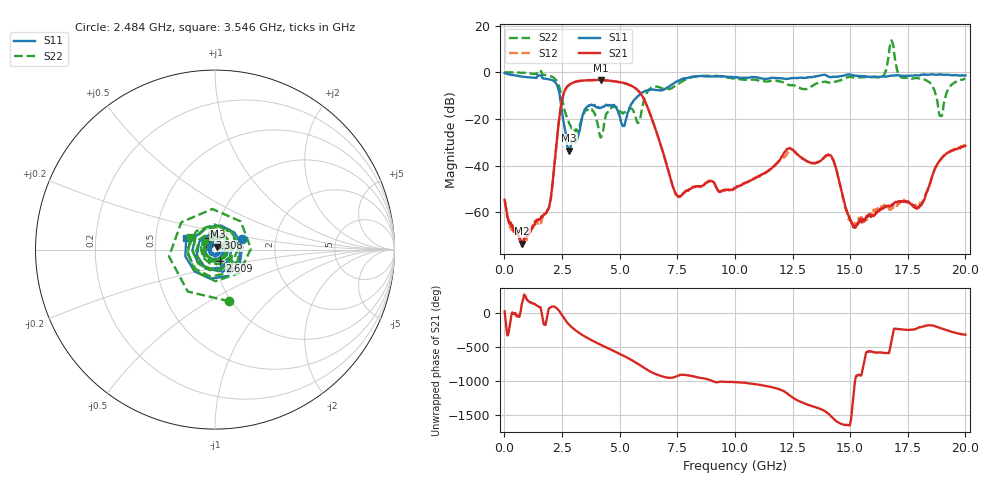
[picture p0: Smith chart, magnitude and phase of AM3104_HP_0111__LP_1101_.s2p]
!Created with skrf (http://scikit-rf.org).
# Hz S RI R 50.0
!freq ReS11 ImS11 ReS21 ImS21 ReS12 ImS12 ReS22 ImS22
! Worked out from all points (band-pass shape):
!   1601 points, 10 MHz to 20 GHz, reference 50 ohm
!   highest |S21| = -3.27 dB at 4.183 GHz (marker M1); lowest = -73.5 dB at 772.1 MHz (marker M2)
!   |S21| within 3 dB of the highest: 2.721 GHz to 5.594 GHz (2.873 GHz wide, 69.1 % of centre)
!   lowest |S11| = -33.7 dB at 2.809 GHz (marker M3), VSWR 1.04, Z = 51.3 + j1.65 ohm
!   |S11| at or under -10 dB: 2.401 GHz to 5.818 GHz (3.417 GHz wide, 83.1 % of centre)
!   |S22| runs from -28.0 to 13.6 dB; largest |S21 - S12| = 0.07
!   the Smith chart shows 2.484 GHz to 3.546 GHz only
!   S11 on the Smith chart (normalised r, x): 2.484 GHz: 1.34, +0.17; 2.609 GHz: 1.04, -0.13; 3.308 GHz: 0.93, +0.12; 3.546 GHz: 0.72, +0.09
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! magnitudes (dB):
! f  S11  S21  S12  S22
! 10 MHz  -0.4  -54.7  -55.3  0.0
! 772.1 MHz  -1.9  -73.5  -74.6  -0.2
! 1.922 GHz  -3.0  -58.3  -58.3  -1.4
! 2.484 GHz  -15.8  -12.8  -12.8  -10.5
! 2.609 GHz  -23.5  -8.1  -8.1  -16.2
! 2.809 GHz  -33.7  -5.4  -5.5  -21.9
! 3.308 GHz  -22.7  -3.7  -3.7  -21.4
! 3.346 GHz  -20.7  -3.6  -3.7  -20.2
! 3.546 GHz  -15.3  -3.5  -3.5  -16.3
! 4.183 GHz  -15.3  -3.3  -3.3  -28.0
! 5.157 GHz  -22.9  -4.5  -4.6  -17.6
! 5.795 GHz  -10.3  -7.8  -7.8  -21.8
! 6.682 GHz  -7.7  -28.1  -28.1  -6.3
! 7.506 GHz  -3.9  -52.9  -53.1  -5.2
! 10.01 GHz  -2.3  -49.8  -49.7  -2.9
! 13.34 GHz  -2.2  -39.0  -39.0  -6.0
! 14.2 GHz  -2.1  -36.4  -36.6  -4.5
! 15.16 GHz  -1.3  -66.5  -64.6  -2.2
! 16.68 GHz  -1.6  -57.5  -58.4  7.3
! 17.99 GHz  -1.3  -57.9  -56.7  -2.7
! 18.93 GHz  -0.8  -37.4  -37.4  -18.8
! 20 GHz  -1.3  -31.6  -31.2  -2.8
